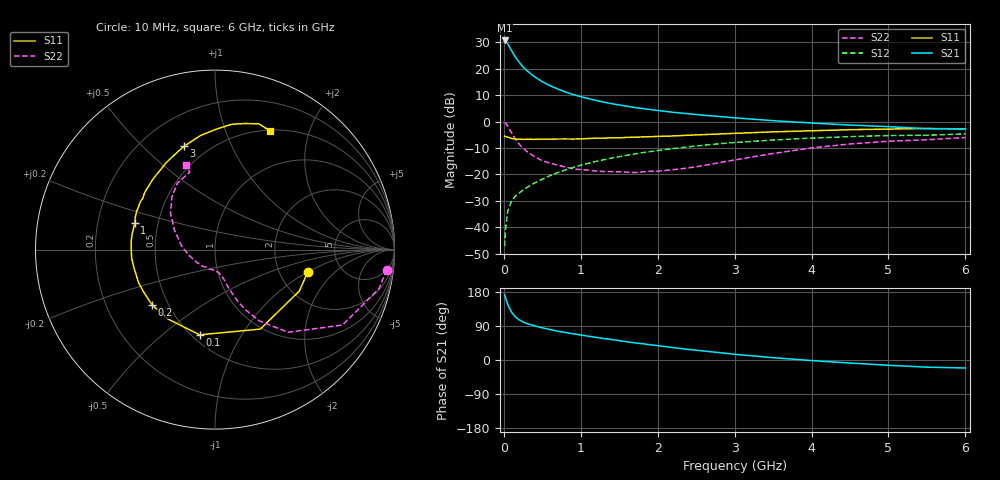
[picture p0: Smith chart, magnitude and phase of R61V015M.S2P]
! SIEMENS Small Signal Semiconductors
! BFR193
! Si NPN RF Bipolar Junction Transistor in SOT23
! VCE = 1 V  IC = 15 mA
! Common Emitter S-Parameters:  May  1996
# GHz  S  MA  R  50
!  f  S11  S21  S12  S22
! GHz  MAG  ANG  MAG  ANG  MAG  ANG  MAG  ANG
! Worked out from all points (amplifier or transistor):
!   36 points, 10 MHz to 6 GHz, reference 50 ohm
!   highest |S21| = 30.7 dB at 10 MHz (marker M1)
!   |S21| within 3 dB of that: start of sweep to 84.74 MHz
!   unconditionally stable (mu >= 1): 584.7 MHz to 2.189 GHz
!   at 250 MHz: K = 0.78, MSG = 23.3 dB, |S12| = -25.9 dB
!   at 1.4 GHz: K = 1.04, MAG = 9.1 dB, |S12| = -13.8 dB
!   at 6 GHz: K = 0.97, MSG = 0.9 dB, |S12| = -4.6 dB
!   S11 on the Smith chart (normalised r, x): 10 MHz: 2.89, -0.99; 100 MHz: 0.55, -0.68; 200 MHz: 0.41, -0.32; 1 GHz: 0.37, +0.14; 3 GHz: 0.37, +0.67; 6 GHz: 0.51, +1.44
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0.01  0.5319 -13.4  34.39 172.8  0.0044 85.9  0.9632 -6.7
0.02  0.5236 -26.1  33.92 165.4  0.0087 79.2  0.9399 -13.3
0.05  0.5097 -60.3  30.06 146.9  0.0199 68.3  0.8255 -30.6
0.1  0.4824 -100.2  22.19 126.3  0.0315 59.4  0.615 -48.5
0.15  0.4673 -124.1  16.79 113.6  0.0389 56.5  0.4682 -58.1
0.2  0.4665 -138.8  13.31 105.9  0.0446 57.1  0.3761 -63.1
0.25  0.4624 -148.9  10.89 100.4  0.0507 57.9  0.3146 -66.2
0.3  0.4638 -156.4  9.23 96.2  0.0567 59.4  0.273 -68.0
0.4  0.4626 -167.3  7.079 90.1  0.0691 61.9  0.2169 -70.9
0.5  0.4668 -174.3  5.701 84.9  0.0816 63.5  0.1826 -72.7
0.6  0.4665 179.3  4.791 80.4  0.0951 64.1  0.1638 -74.1
0.7  0.4694 174.1  4.151 76.2  0.1083 64.2  0.15 -76.3
0.8  0.4698 169.4  3.65 72.5  0.1219 64.1  0.1381 -78.9
1  0.4711 161.4  2.969 65.9  0.1495 63.3  0.1237 -84.2
1.1  0.4797 157.7  2.722 62.7  0.1632 62.4  0.121 -88.0
1.6  0.5034 141.4  1.95 48.1  0.2308 56.9  0.1108 -110.7
2.2  0.536 125.1  1.503 32.8  0.3095 48.8  0.1234 -144.5
3  0.6008 106.7  1.183 15.1  0.4032 36.4  0.1882 173.2
3.5  0.6405 97.3  1.043 6.2  0.449 28.5  0.2496 154.5
4.5  0.705 82.3  0.862 -8.0  0.5213 14.1  0.3779 129.5
5.5  0.7423 70.6  0.734 -18.9  0.5532 0.1  0.4538 108.0
6  0.7288 65.2  0.724 -21.1  0.5869 -4.1  0.4997 108.8
